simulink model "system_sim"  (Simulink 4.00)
settings: Solver=FixedStepDiscrete  SolverMode=SingleTasking  StartTime=0.0  StopTime=500  FixedStep=1  RelTol=1e-3  AbsTol=1e-6
PostLoadFcn:
  | system_postloadfcn
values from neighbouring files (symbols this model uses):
  w = 0.1    [system_postloadfcn.m]
libraries: labmvlib x3

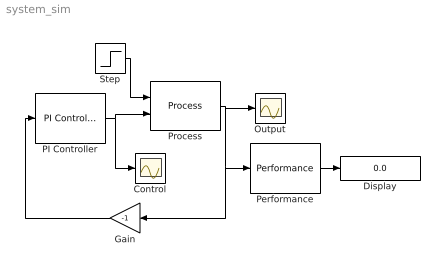
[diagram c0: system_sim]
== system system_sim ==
  Control : Scope
  Display : Display
  Gain : Gain  Orientation=left  Gain=-1  Multiplication=Element-wise(K.*u)  SaturateOnIntegerOverflow=on
  Output : Scope
  PI Controller : labmvlib/PI Controller
  Performance : labmvlib/Performance
  Process : labmvlib/Process
  Step : Step  Time=250  Before=w  After=10*w  SampleTime=1
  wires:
  Process/1 -> Output/1, Gain/1, Performance/1
  Performance/1 -> Display/1
  Step/1 -> Process/1
  Gain/1 -> PI Controller/1
  PI Controller/1 -> Control/1, Process/2
